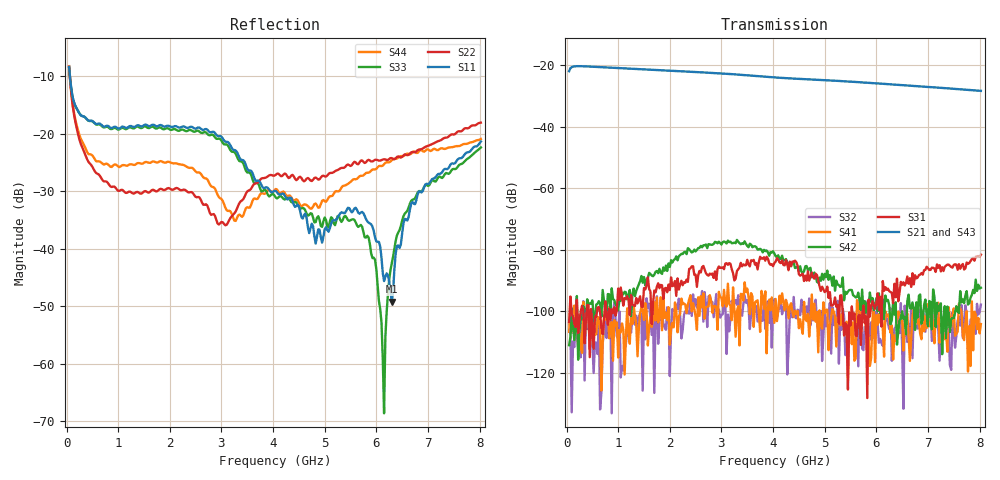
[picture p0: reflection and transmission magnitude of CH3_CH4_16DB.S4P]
!Agilent Technologies,E5071C,MY46316741,A.11.02
!Date: Thu May 28 15:02:28 2026
!Data & Calibration Information:
!1:CH3 INPUT 2:CH3 OUTPUT 3:CH4 INPUT 4:CH4 OUTPUT
!Freq	S11:SOLT4(ON)	S12:SOLT4(ON)	S13:SOLT4(ON)	S14:SOLT4(ON)
!	S21:SOLT4(ON)	S22:SOLT4(ON)	S23:SOLT4(ON)	S24:SOLT4(ON)
!	S31:SOLT4(ON)	S32:SOLT4(ON)	S33:SOLT4(ON)	S34:SOLT4(ON)
!	S41:SOLT4(ON)	S42:SOLT4(ON)	S43:SOLT4(ON)	S44:SOLT4(ON)
!PortZ  Port1:50+j0  Port2:50+j0  Port3:50+j0  Port4:50+j0
!Above PortZ is port z conversion or system Z0 setting when saving the data.
!When reading, reference impedance value at option line is always used.
# Hz S dB R 50
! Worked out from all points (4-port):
!   320 points, 50 MHz to 8.025 GHz, reference 50 ohm
!   strongest paths, dB at 50 MHz, 2.05 GHz, 4.05 GHz, 6.05 GHz, 8.025 GHz:
!     S21: -22.0, -21.8, -24.0, -26.0, -28.3
!     S43: -21.8, -21.8, -24.0, -26.0, -28.5
!     S31: -103.4, -91.8, -83.8, -99.6, -81.6
!     S42: -111.0, -84.1, -82.1, -94.2, -92.3
!     S41: -106.7, -103.8, -96.0, -100.9, -104.1
!     S32: -102.8, -99.3, -99.1, -110.2, -97.8
!   lowest |S11| = -49.2 dB at 6.3 GHz (marker M1), VSWR 1.01, Z = 50 + j0.345 ohm
!   |S11| at or under -10 dB: 65.79 MHz to end of sweep
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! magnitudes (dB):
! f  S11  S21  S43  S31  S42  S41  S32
! 50 MHz  -8.4  -22.0  -21.8  -103.4  -111.0  -106.7  -102.8
! 2.95 GHz  -20.4  -22.6  -22.6  -85.4  -77.4  -93.7  -99.3
! 5.7 GHz  -33.7  -25.6  -25.6  -110.9  -99.7  -103.1  -95.8
! 6 GHz  -38.7  -25.9  -26.0  -97.5  -95.8  -101.2  -100.0
! 6.15 GHz  -45.6  -26.1  -26.2  -93.3  -102.6  -114.7  -107.1
! 6.3 GHz  -49.2  -26.2  -26.3  -94.0  -102.8  -104.6  -116.1
! 8.025 GHz  -21.4  -28.3  -28.5  -81.6  -92.3  -104.1  -97.8
